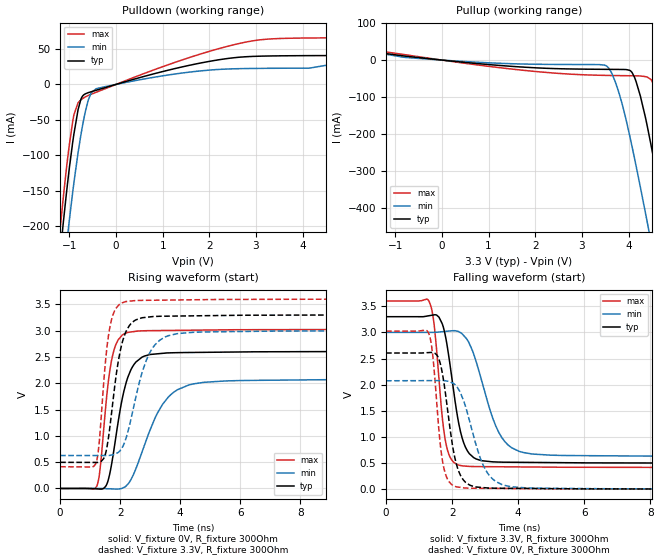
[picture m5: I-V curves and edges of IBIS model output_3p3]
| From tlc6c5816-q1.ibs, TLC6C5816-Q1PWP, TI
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|   output_3p3 Model
[Model]   output_3p3
Model_type   Output
Polarity   Non-Inverting
Vmeas = 1.65
Vref = 0
Cref = 2pF
Rref = 100000
|   typ   min   max
C_comp   2.702pF   2.604pF   2.816pF
|  Where Nom  PVT is Nominal Process, 3.3V,  27C
|   Fast PVT is Strong Process,  3.6V, -40C
|   Slow PVT is Weak Process,   3.0V, 150C
[Voltage Range]   3.3   3   3.6
|Junction Temperature
[Temperature Range]   27   150   -40
[Pullup Reference]   3.3   3   3.6
[Pulldown Reference]   0   0   0
[Power Clamp Reference]   3.3   3   3.6
[GND Clamp Reference]   0   0   0
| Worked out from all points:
|   slope of the pulldown table from 0 to 0.495 V, typ, clamps not added: 53.2 ohm
|   slope of the pullup table from 0 to 0.495 V, typ, clamps not added: 78.5 ohm
|   falling waveform, V_fixture 3.3V, R_fixture 300Ohm: 20-80 % time 420ps typ, 718ps min, 278ps max; typ from 3.3 V to 0.497 V
|   rising waveform, V_fixture 0V, R_fixture 300Ohm: 20-80 % time 506ps typ, 945ps min, 335ps max; typ from 0 V to 2.6 V
|   rising waveform, V_fixture 3.3V, R_fixture 300Ohm: 20-80 % time 421ps typ, 672ps min, 298ps max; typ from 0.497 V to 3.3 V
|   falling waveform, V_fixture 0V, R_fixture 300Ohm: 20-80 % time 373ps typ, 610ps min, 257ps max; typ from 2.6 V to 0 V
[Pulldown]
|   Voltage   I(typ)   I(min)   I(max)
-3.3V     -1.769A    -1.731A    -1.808A
-1.28V    -292.8mA   -360.3mA   -260.3mA
-1.171V   -219.8mA   -291.8mA   -184.8mA
-1.132V   -194.3mA   -267.4mA   -158.8mA
-1.013V   -123.4mA   -197mA     -90.04mA
-904.2mV  -69.56mA   -137.9mA   -42.63mA
-755.7mV  -21mA      -71.44mA   -21.89mA
-656.7mV  -13.23mA   -37.55mA   -17.48mA
-399.3mV  -7.742mA   -5.625mA   -10.37mA
2.788V    38.91mA    22.28mA    59.6mA
5.362V    41.88mA    45.81mA    65.7mA
6.6V      76.24mA    78.99mA    76.45mA
[Pullup]
|   Voltage   I(typ)   I(min)   I(max)
-3.3V     74.78mA    69.94mA    83.58mA
-815.1mV  11.11mA    7.531mA    14.96mA
3.482V    -25.01mA   -13.5mA    -41.34mA
3.709V    -25.21mA   -56.52mA   -41.83mA
4.026V    -27.77mA   -204.8mA   -42.35mA
4.165V    -59.01mA   -287.6mA   -42.56mA
4.402V    -178.5mA   -438.6mA   -46.03mA
4.561V    -281.3mA   -542.5mA   -75.93mA
4.778V    -432.4mA   -687.8mA   -195.1mA
4.986V    -580.8mA   -828.1mA   -341.3mA
5.303V    -810.7mA   -1.044A    -577.7mA
6.6V      -1.768A    -1.939A    -1.576A
[Ramp]
R_load = 300
|   typ   min   max
dV/dt_r   1.56312/5.06442e-10   1.24429/9.38405e-10   1.81414/3.35495e-10
dV/dt_f   1.68193/4.19793e-10   1.42416/7.17561e-10   1.9119/2.77761e-10
[Falling Waveform]
V_fixture = 3.3V
V_fixture_min = 3V
V_fixture_max = 3.6V
R_fixture = 300Ohm
C_fixture = 0F
|   Time   V(typ)   V(min)   V(max)
0s        3.3V       3V         3.6V
1.309ns   3.319V     3V         3.587V
1.451ns   3.335V     3V         3.173V
1.603ns   3.29V      3.007V     2.104V
1.895ns   2.564V     3.024V     678.9mV
2.207ns   1.238V     3.012V     460.6mV
2.485ns   712.4mV    2.831V     436.6mV
3.504ns   517mV      988.3mV    428.3mV
4.994ns   508.8mV    650.3mV    421.1mV
100ns     496.8mV    626.4mV    413.5mV
[Rising Waveform]
V_fixture = 0V
V_fixture_min = 0V
V_fixture_max = 0V
R_fixture = 300Ohm
C_fixture = 0F
|   Time   V(typ)   V(min)   V(max)
0s        -74.02nV   -338.1nV   -235.2nV
1.213ns   -7.057mV   178.8uV    36.61mV
1.344ns   -12.35mV   198.1uV    441.7mV
1.535ns   58.01mV    -3.887mV   1.657V
1.858ns   984.7mV    -11.55mV   2.738V
2.207ns   2.028V     51.46mV    2.957V
2.599ns   2.437V     487.1mV    2.993V
3.696ns   2.578V     1.788V     3.004V
5.81ns    2.593V     2.048V     3.017V
100ns     2.605V     2.074V     3.024V
[Rising Waveform]
V_fixture = 3.3V
V_fixture_min = 3V
V_fixture_max = 3.6V
R_fixture = 300Ohm
C_fixture = 0F
|   Time   V(typ)   V(min)   V(max)
0s        496.8mV    626.4mV    413.5mV
1.177ns   494.7mV    626.2mV    460.3mV
1.297ns   501mV      626.2mV    844.1mV
1.449ns   567.7mV    626.2mV    1.991V
1.763ns   1.675V     641.5mV    3.305V
2.086ns   2.809V     795.7mV    3.532V
2.485ns   3.192V     1.639V     3.571V
3.162ns   3.269V     2.732V     3.578V
4.783ns   3.284V     2.974V     3.589V
100ns     3.3V       3V         3.6V
[Falling Waveform]
|Gnd
V_fixture = 0V
V_fixture_min = 0V
V_fixture_max = 0V
R_fixture = 300Ohm
C_fixture = 0F
|   Time   V(typ)   V(min)   V(max)
0s        2.605V     2.074V     3.024V
1.282ns   2.613V     2.077V     2.995V
1.404ns   2.614V     2.077V     2.615V
1.577ns   2.523V     2.077V     1.306V
1.763ns   1.99V      2.076V     370.3mV
2.086ns   591.9mV    2.001V     55.33mV
2.39ns    142mV      1.614V     22.35mV
3.162ns   20.71mV    235.5mV    15.56mV
4.428ns   12.96mV    20.24mV    9.712mV
100ns     -74.03nV   -581.1nV   -239.1nV
